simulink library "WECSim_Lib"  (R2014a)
settings: Solver=ode45  StartTime=0.0  StopTime=10.0  RelTol=1e-3
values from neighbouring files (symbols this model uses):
  geometry = 'NOT DEFINED'    [bodyClass.m]
  m = plot(Rel.WEC_Sim_org.time(find(Rel.WEC_Sim_org.time==350):end),     Rel.WEC_Sim_org.heave(find(Rel.WEC_Sim_org.time==350):end),'r-',     Rel.WEC_Sim_new.time(find(Rel.WEC_Sim_new.time==350):end),     Rel.WEC_Sim_new.heave(find(Rel.WEC_Sim_new.time==350):end),'k-')    [runTestCase.m]
  simu = simulationClass    [wecSim.m]
  waves = waveClass(waves.type,0,0,simu,'Imported',waves.randPreDefined,waves.spectrumDataFile)    [waveSetup.m]
undefined symbols (not defined in the file or in its folder): body, constraint, deg, flap, kg, N, pto, rad, s, X, Y, Z
libraries: nesl_utility x41, sm_lib x30
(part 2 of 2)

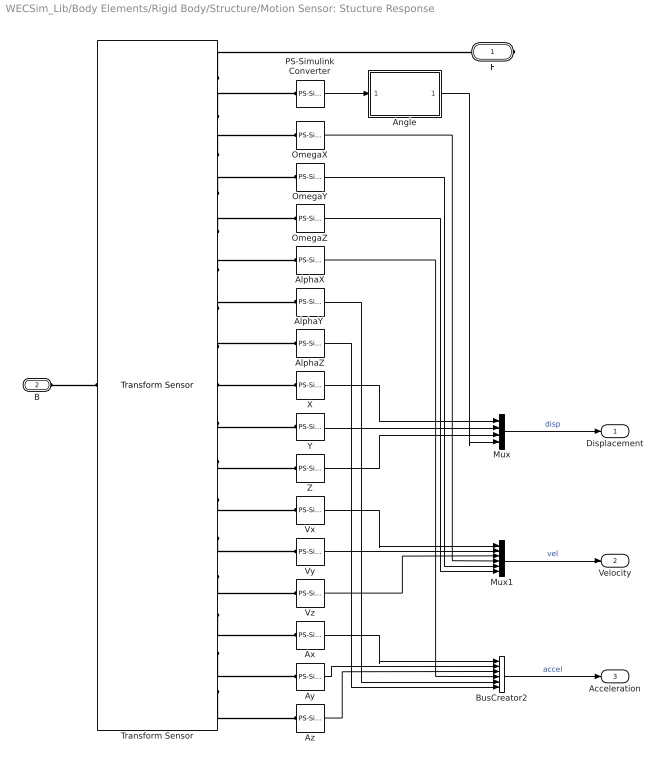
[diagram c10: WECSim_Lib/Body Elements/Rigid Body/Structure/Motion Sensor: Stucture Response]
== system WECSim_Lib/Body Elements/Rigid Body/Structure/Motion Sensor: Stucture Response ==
  AlphaX : nesl_utility/PS-Simulink Converter  PhysicalDomain=network_engine_domain  SubClassName=ps_output  LeftPortType=input  RightPortType=output  PseudoPeriodic=off  Frequencies=[]  Unit=1  AffineConversion=off
  "AlphaY " : nesl_utility/PS-Simulink Converter  PhysicalDomain=network_engine_domain  SubClassName=ps_output  LeftPortType=input  RightPortType=output  PseudoPeriodic=off  Frequencies=[]  Unit=1  AffineConversion=off
  AlphaZ : nesl_utility/PS-Simulink Converter  PhysicalDomain=network_engine_domain  SubClassName=ps_output  LeftPortType=input  RightPortType=output  PseudoPeriodic=off  Frequencies=[]  Unit=1  AffineConversion=off
  Angle : MATLAB Function  TreatAsAtomicUnit=on
  Ax : nesl_utility/PS-Simulink Converter  PhysicalDomain=network_engine_domain  SubClassName=ps_output  LeftPortType=input  RightPortType=output  PseudoPeriodic=off  Frequencies=[]  Unit=1  AffineConversion=off
  Ay : nesl_utility/PS-Simulink Converter  PhysicalDomain=network_engine_domain  SubClassName=ps_output  LeftPortType=input  RightPortType=output  PseudoPeriodic=off  Frequencies=[]  Unit=1  AffineConversion=off
  Az : nesl_utility/PS-Simulink Converter  PhysicalDomain=network_engine_domain  SubClassName=ps_output  LeftPortType=input  RightPortType=output  PseudoPeriodic=off  Frequencies=[]  Unit=1  AffineConversion=off
  BusCreator2 : BusCreator  Inputs=6
  Mux : Mux
  Mux1 : Mux  Inputs=6
  OmegaX : nesl_utility/PS-Simulink Converter  PhysicalDomain=network_engine_domain  SubClassName=ps_output  LeftPortType=input  RightPortType=output  PseudoPeriodic=off  Frequencies=[]  Unit=1  AffineConversion=off
  OmegaY : nesl_utility/PS-Simulink Converter  PhysicalDomain=network_engine_domain  SubClassName=ps_output  LeftPortType=input  RightPortType=output  PseudoPeriodic=off  Frequencies=[]  Unit=1  AffineConversion=off
  OmegaZ : nesl_utility/PS-Simulink Converter  PhysicalDomain=network_engine_domain  SubClassName=ps_output  LeftPortType=input  RightPortType=output  PseudoPeriodic=off  Frequencies=[]  Unit=1  AffineConversion=off
  PS-Simulink Converter : nesl_utility/PS-Simulink Converter  PhysicalDomain=network_engine_domain  SubClassName=ps_output  LeftPortType=input  RightPortType=output  PseudoPeriodic=off  Frequencies=[]  Unit=1  AffineConversion=off
  Transform Sensor : sm_lib/Frames and Transforms/Transform Sensor  MeasurementFrame=World  SenseAngle=off  SenseAxis=off  SenseAngle1=off  SenseAngle2=off  SenseAngle3=off  SenseQ=on  SenseR=off  SenseOmegaX=on  SenseOmegaY=on  SenseOmegaZ=on  SenseOmega1=off  SenseOmega2=off  SenseOmega3=off  SenseQDot=off  SenseRDot=off  SenseAlphaX=on  SenseAlphaY=on  SenseAlphaZ=on  SenseAlpha1=off  SenseAlpha2=off  SenseAlpha3=off  SenseQDDot=off  SenseRDDot=off  SenseX=on  SenseY=on  SenseZ=on  SenseRad=off  SenseAzim=off  SenseDist=off  SenseInc=off  SenseXDot=on  SenseYDot=on  SenseZDot=on  SenseRadDot=off  SenseAzimDot=off  SenseDistDot=off  SenseIncDot=off  SenseXDDot=on  SenseYDDot=on  SenseZDDot=on  SenseRadDDot=off  SenseAzimDDot=off  SenseDistDDot=off  SenseIncDDot=off  BlockFunction=simmechanics.library.frames_transforms.transform_sensor
  Vx : nesl_utility/PS-Simulink Converter  PhysicalDomain=network_engine_domain  SubClassName=ps_output  LeftPortType=input  RightPortType=output  PseudoPeriodic=off  Frequencies=[]  Unit=1  AffineConversion=off
  Vy : nesl_utility/PS-Simulink Converter  PhysicalDomain=network_engine_domain  SubClassName=ps_output  LeftPortType=input  RightPortType=output  PseudoPeriodic=off  Frequencies=[]  Unit=1  AffineConversion=off
  Vz : nesl_utility/PS-Simulink Converter  PhysicalDomain=network_engine_domain  SubClassName=ps_output  LeftPortType=input  RightPortType=output  PseudoPeriodic=off  Frequencies=[]  Unit=1  AffineConversion=off
  X : nesl_utility/PS-Simulink Converter  PhysicalDomain=network_engine_domain  SubClassName=ps_output  LeftPortType=input  RightPortType=output  PseudoPeriodic=off  Frequencies=[]  Unit=1  AffineConversion=off
  Y : nesl_utility/PS-Simulink Converter  PhysicalDomain=network_engine_domain  SubClassName=ps_output  LeftPortType=input  RightPortType=output  PseudoPeriodic=off  Frequencies=[]  Unit=1  AffineConversion=off
  Z : nesl_utility/PS-Simulink Converter  PhysicalDomain=network_engine_domain  SubClassName=ps_output  LeftPortType=input  RightPortType=output  PseudoPeriodic=off  Frequencies=[]  Unit=1  AffineConversion=off
  F : PMIOPort  Port=1  Side=Right
  B : PMIOPort  Port=2  Side=Left
  Displacement : Outport
  Velocity : Outport  Port=2
  Acceleration : Outport  Port=3
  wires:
  PS-Simulink Converter/1 -> Angle/1(Q)
  AlphaX/1 -> BusCreator2/4
  Vx/1 -> Mux1/1
  Vy/1 -> Mux1/2
  Vz/1 -> Mux1/3
  Ax/1 -> BusCreator2/1
  Ay/1 -> BusCreator2/2
  Az/1 -> BusCreator2/3
  Mux/1 -> Displacement/1  "disp"
  Mux1/1 -> Velocity/1  "vel"
  BusCreator2/1 -> Acceleration/1  "accel"
  Angle/1(E) -> Mux/4
  X/1 -> Mux/1
  Y/1 -> Mux/2
  Z/1 -> Mux/3
  "AlphaY "/1 -> BusCreator2/5
  AlphaZ/1 -> BusCreator2/6
  OmegaX/1 -> Mux1/4
  OmegaY/1 -> Mux1/5
  OmegaZ/1 -> Mux1/6
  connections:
  Transform Sensor/RConn1 -- F/RConn1
  B/RConn1 -- Transform Sensor/LConn1
  Transform Sensor/RConn2 -- PS-Simulink Converter/LConn1
  Transform Sensor/RConn17 -- Az/LConn1
  Transform Sensor/RConn16 -- Ay/LConn1
  Transform Sensor/RConn15 -- Ax/LConn1
  Transform Sensor/RConn14 -- Vz/LConn1
  Transform Sensor/RConn13 -- Vy/LConn1
  Transform Sensor/RConn12 -- Vx/LConn1
  Transform Sensor/RConn11 -- Z/LConn1
  Transform Sensor/RConn10 -- Y/LConn1
  Transform Sensor/RConn9 -- X/LConn1
  Transform Sensor/RConn6 -- AlphaX/LConn1
  Transform Sensor/RConn7 -- "AlphaY "/LConn1
  Transform Sensor/RConn8 -- AlphaZ/LConn1
  Transform Sensor/RConn3 -- OmegaX/LConn1
  Transform Sensor/RConn4 -- OmegaY/LConn1
  Transform Sensor/RConn5 -- OmegaZ/LConn1

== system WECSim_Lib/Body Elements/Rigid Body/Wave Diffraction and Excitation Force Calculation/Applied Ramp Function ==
  In1 : Inport
  Action Port : ActionPort  ActionType=then
  Add : Sum
  Constant : Constant  Value=2
  Constant1 : Constant
  Divide : Product  Inputs=**/
  Sine Wave : Sin  Frequency=pi/simu.rampT  Phase=pi+pi/2  SampleTime=0
  Out1 : Outport
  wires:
  Add/1 -> Divide/2
  Sine Wave/1 -> Add/2
  Constant1/1 -> Add/1
  Constant/1 -> Divide/3
  Divide/1 -> Out1/1
  In1/1 -> Divide/1

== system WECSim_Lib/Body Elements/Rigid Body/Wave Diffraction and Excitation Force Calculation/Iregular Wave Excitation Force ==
  Time : Inport
  Action Port : ActionPort  ActionType=else
  Excitation Re Part2 : Constant  Value=body.hydroForce.fExt.re  VectorParams1D=off
  Excitation Re Part3 : Constant  Value=body.hydroForce.fExt.im  VectorParams1D=off
  For Each Subsystem : Subsystem  TreatAsAtomicUnit=on
  Sum of Elements : Sum  Inputs=+  CollapseMode=Specified dimension
  dw1 : Constant  Value=(waves.w(end)-waves.w(1))/(waves.numFreq-1)  VectorParams1D=off
  wave frequency : Constant  Value=waves.w  VectorParams1D=off
  wave frequency1 : Constant  Value=waves.phaseRand'  VectorParams1D=off
  wave spectrum : Constant  Value=waves.A*2  VectorParams1D=off
  F_wave : Outport  PortDimensions=6
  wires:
  dw1/1 -> For Each Subsystem/6(dw)
  wave frequency1/1 -> For Each Subsystem/7(phaseRand)
  Sum of Elements/1 -> F_wave/1
  Time/1 -> For Each Subsystem/5(Time)
  For Each Subsystem/1(Out1) -> Sum of Elements/1
  wave spectrum/1 -> For Each Subsystem/1(wave amplitude)
  wave frequency/1 -> For Each Subsystem/2(wave freq)
  Excitation Re Part3/1 -> For Each Subsystem/4(wave fExt im)
  Excitation Re Part2/1 -> For Each Subsystem/3(wave fExt re)

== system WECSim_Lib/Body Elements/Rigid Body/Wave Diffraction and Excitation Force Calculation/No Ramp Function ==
  In1 : Inport
  Action Port : ActionPort  ActionType=else
  Out1 : Outport
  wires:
  In1/1 -> Out1/1

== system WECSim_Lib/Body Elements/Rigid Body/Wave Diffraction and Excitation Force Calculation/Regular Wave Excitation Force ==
  Action Port : ActionPort  ActionType=then
  Add : Sum  Inputs=+-
  Cos Wave : Sin  Amplitude=waves.A(1,:)  Frequency=waves.w(1,:)  Phase=pi/2  SampleTime=0
  Product : Product  Inputs=**
  Product1 : Product  Inputs=**
  Sin Wave : Sin  Amplitude=waves.A(1,:)  Frequency=waves.w(1,:)  SampleTime=0
  WAMIT Excitation Im Part1 : Constant  Value=body.hydroForce.fExt.im(1,:)  VectorParams1D=off
  WAMIT Excitation Re Part : Constant  Value=body.hydroForce.fExt.re(1,:)  VectorParams1D=off
  F_wave : Outport  PortDimensions=6
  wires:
  Add/1 -> F_wave/1
  Product/1 -> Add/1
  WAMIT Excitation Im Part1/1 -> Product1/2
  Product1/1 -> Add/2
  Sin Wave/1 -> Product1/1
  WAMIT Excitation Re Part/1 -> Product/2
  Cos Wave/1 -> Product/1

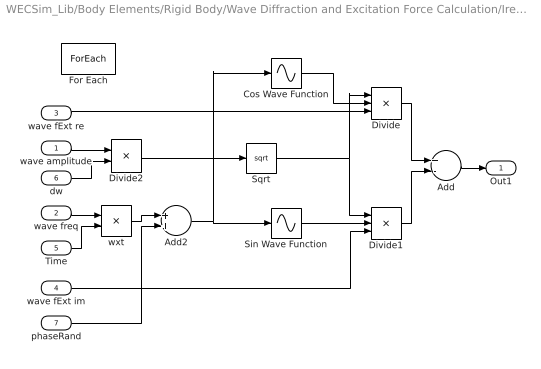
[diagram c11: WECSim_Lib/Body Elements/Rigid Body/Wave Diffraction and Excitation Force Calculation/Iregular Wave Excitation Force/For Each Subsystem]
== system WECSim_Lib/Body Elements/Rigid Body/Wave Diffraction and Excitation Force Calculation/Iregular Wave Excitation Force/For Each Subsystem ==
  wave amplitude : Inport  Partition=on  PartitionDimension=1  PartitionWidth=1
  wave freq : Inport  Port=2  Partition=on  PartitionDimension=1  PartitionWidth=1
  wave fExt re : Inport  Port=3  Partition=on  PartitionDimension=1  PartitionWidth=1
  wave fExt im : Inport  Port=4  Partition=on  PartitionDimension=1  PartitionWidth=1
  Time : Inport  Port=5  Partition=off
  dw : Inport  Port=6  Partition=off
  phaseRand : Inport  Port=7  Partition=on  PartitionDimension=1  PartitionWidth=1
  Add : Sum  Inputs=+-
  Add2 : Sum
  Cos Wave Function : Sin  TimeSource=Use external signal  Phase=pi/2  SampleTime=0
  Divide : Product  Inputs=***
  Divide1 : Product  Inputs=***
  Divide2 : Product  Inputs=**
  For Each : ForEach  DisableCoverage=on  IndexMode=One-based
  Sin Wave Function : Sin  TimeSource=Use external signal  SampleTime=0
  Sqrt : Sqrt
  wxt : Product  Inputs=**
  Out1 : Outport  ConcatenationDimension=1
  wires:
  Add2/1 -> Cos Wave Function/1, Sin Wave Function/1
  phaseRand/1 -> Add2/2
  wxt/1 -> Add2/1
  Sqrt/1 -> Divide/1, Divide1/1
  Divide2/1 -> Sqrt/1
  dw/1 -> Divide2/2
  wave amplitude/1 -> Divide2/1
  Time/1 -> wxt/2
  Add/1 -> Out1/1
  Cos Wave Function/1 -> Divide/2
  wave fExt re/1 -> Divide/3
  wave freq/1 -> wxt/1
  Sin Wave Function/1 -> Divide1/2
  wave fExt im/1 -> Divide1/3
  Divide/1 -> Add/1
  Divide1/1 -> Add/2
